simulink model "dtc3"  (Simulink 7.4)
settings: Solver=ode45  StartTime=0.0  StopTime=2  MaxStep=5e-6  RelTol=1e-3
InitFcn:
  | warning off; wmo=0.9 %initial speed
  | fso=1.0 %initial stator flux
undefined symbols (not defined in the file or in its folder): a, wmo

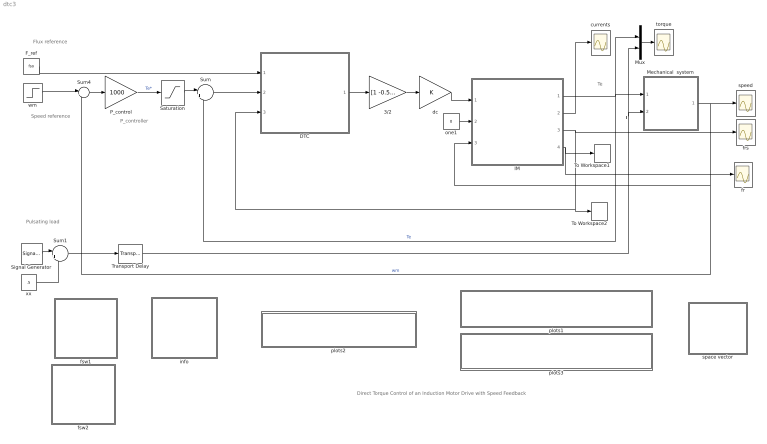
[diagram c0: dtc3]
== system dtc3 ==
  note: Direct Torque Control of an Induction Motor Drive with Speed Feedback
  note: Flux reference
  note: Speed reference
  note: Te
  note: Tl
  note: Pulsating load
  note: P_controller
  3/2 : Gain  Gain=[1 -0.5 -0.5;0 sqrt(3)/2 -sqrt(3)/2]  Multiplication=Matrix(K*u)  ParameterDataType=sfix(16)  ParameterScaling=2^0  OutDataType=sfix(16)  OutScaling=2^0
  DTC : Subsystem
  F_ref : Constant  Value=fso  OutDataType=sfix(16)  OutScaling=2^0
  IM : Subsystem  mask{Rs=0.01, Rr=0.02, Lsl=0.10, Lrl=0.10, Lm=4.5, wo=2*pi*60}
      mask prompts: Rs "Stator resistance [pu]"; Rr "Rotor resistance [pu]"; Lsl "Stator leakage inductance [pu]"; Lrl "Rotor leakage inductance [pu]"; Lm "Magnetizing inductance [pu]"; wo "Base frequency [rad/s]"
  Mechanical  system : Subsystem  mask{H=0.5, Bm=1e-5}
      mask prompts: H "Inertia constant [s]"; Bm "Torque-speed coefficient"
  Mux : Mux  Inputs=2
  P_control : Gain  Gain=1000  ParameterDataType=sfix(16)  ParameterScaling=2^0  OutDataType=sfix(16)  OutScaling=2^0
  Saturation : Saturate  UpperLimit=2  LowerLimit=-2
  Signal Generator : SignalGenerator  WaveForm=square  Amplitude=.5  Frequency=4
  Sum : Sum  Inputs=|+-  OutDataType=sfix(16)  OutScaling=2^0
  Sum1 : Sum  Inputs=|++  OutDataType=sfix(16)  OutScaling=2^0
  Sum4 : Sum  Inputs=|+-  OutDataType=sfix(16)  OutScaling=2^0
  To Workspace1 : ToWorkspace  VariableName=fr  SampleTime=-1  SaveFormat=Array
  To Workspace2 : ToWorkspace  VariableName=fs  SampleTime=-1  SaveFormat=Array
  Transport Delay : TransportDelay  DelayTime=.75
  currents : Scope
  dc : Gain  ParameterDataType=sfix(16)  ParameterScaling=2^0  OutDataType=sfix(16)  OutScaling=2^0
  fr : Scope
  frs : Scope
  fsw1 : Subsystem
  fsw2 : Subsystem
  info : Subsystem
  one1 : Constant  Value=0  OutDataType=sfix(16)  OutScaling=2^0
  plots1 : Subsystem
  plots2 : Subsystem
  plots3 : Subsystem
  space vector : Subsystem
  speed : Scope
  torque : Scope
  wm : Step  Time=.25  Before=wmo  After=.5  SampleTime=0
  xx : Constant  Value=.5  OutDataType=sfix(16)  OutScaling=2^0
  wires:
  DTC/1(s3) -> 3/2/1
  F_ref/1 -> DTC/1(f_ref)
  3/2/1 -> dc/1
  IM/3(fs) -> To Workspace2/1, DTC/3(fs), frs/1
  one1/1 -> IM/2(wk)
  IM/1(Te) -> Mechanical  system/1(Te), Sum/2, Mux/1  "Te"
  Mechanical  system/1(wm) -> speed/1, IM/3(wm), Sum4/2  "wm"
  IM/2(is) -> currents/1
  wm/1 -> Sum4/1
  Sum/1 -> DTC/2(T_er)
  Mux/1 -> torque/1
  Sum4/1 -> P_control/1
  P_control/1 -> Saturation/1  "Te*"
  IM/4(fr) -> To Workspace1/1, fr/1
  dc/1 -> IM/1(vs)
  Signal Generator/1 -> Sum1/1
  xx/1 -> Sum1/2
  Sum1/1 -> Transport Delay/1
  Transport Delay/1 -> Mux/2, Mechanical  system/2(Tl)
  Saturation/1 -> Sum/1

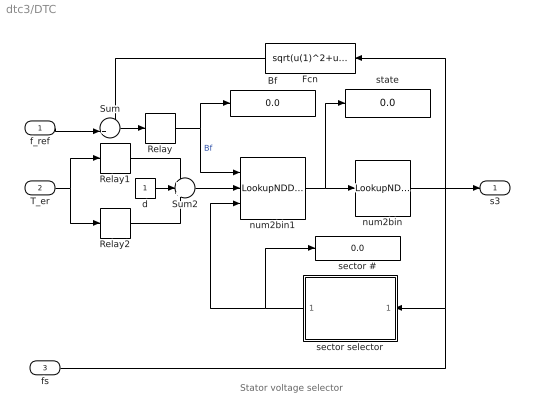
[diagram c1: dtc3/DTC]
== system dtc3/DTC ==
  note: Stator voltage selector
  f_ref : Inport  OutDataType=sfix(16)  OutScaling=2^0
  T_er : Inport  Port=2  OutDataType=sfix(16)  OutScaling=2^0
  fs : Inport  Port=3  OutDataType=sfix(16)  OutScaling=2^0
  Bf : Display
  Fcn : Fcn  Expr=sqrt(u(1)^2+u(2)^2)
  Relay : Relay  OnSwitchValue=.01  OffSwitchValue=-.01  OutDataType=sfix(16)  OutScaling=2^0
  Relay1 : Relay  OnSwitchValue=.02  OffSwitchValue=0  OutDataType=sfix(16)  OutScaling=2^0
  Relay2 : Relay  OnSwitchValue=0  OffSwitchValue=-.02  OnOutputValue=0  OffOutputValue=-1  OutDataType=sfix(16)  OutScaling=2^0
  Sum : Sum  Inputs=-+|  OutDataType=sfix(16)  OutScaling=2^0
  Sum2 : Sum  Inputs=+++  OutDataType=sfix(16)  OutScaling=2^0
  d : Constant  OutDataType=sfix(16)  OutScaling=2^0
  num2bin : LookupNDDirect  InputsSelectThisObjectFromTable=Column  Table=[0 0 0;1 0 0;0 1 0;1 1 0;0 0 1;1 0 1;0 1 1;1 1 1]'  ActionForOutOfRangeInput=Error
  num2bin1 : LookupNDDirect  NumberOfTableDimensions=3  Table=a  ActionForOutOfRangeInput=Error
  sector # : Display
  sector selector : Subsystem
  state : Display
  s3 : Outport
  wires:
  num2bin1/1 -> state/1, num2bin/1
  Sum/1 -> Relay/1
  Relay/1 -> Bf/1, num2bin1/1  "Bf"
  Fcn/1 -> Sum/1
  Sum2/1 -> num2bin1/2
  Relay1/1 -> Sum2/1
  Relay2/1 -> Sum2/3
  d/1 -> Sum2/2
  T_er/1 -> Relay2/1, Relay1/1
  f_ref/1 -> Sum/2
  num2bin/1 -> s3/1
  fs/1 -> Fcn/1, sector selector/1(fs)
  sector selector/1(sector) -> num2bin1/3, sector #/1

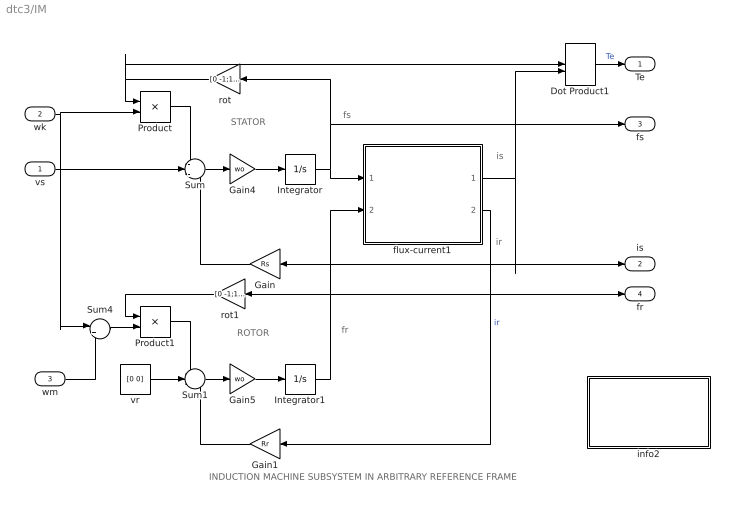
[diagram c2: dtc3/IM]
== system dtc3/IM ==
  note: ROTOR
  note: STATOR
  note: fs
  note: fr
  note: is
  note: INDUCTION MACHINE SUBSYSTEM IN ARBITRARY REFERENCE FRAME
  note: ir
  vs : Inport  OutDataType=sfix(16)  OutScaling=2^0
  wk : Inport  Port=2  OutDataType=sfix(16)  OutScaling=2^0
  wm : Inport  Port=3  OutDataType=sfix(16)  OutScaling=2^0
  Dot Product1 : DotProduct  OutDataType=fixdt(1, 16)  OutScaling=2^-10
  Gain : Gain  Gain=Rs  ParameterDataType=sfix(16)  ParameterScaling=2^0  OutDataType=sfix(16)  OutScaling=2^0
  Gain1 : Gain  Gain=Rr  ParameterDataType=sfix(16)  ParameterScaling=2^0  OutDataType=sfix(16)  OutScaling=2^0
  Gain4 : Gain  Gain=wo  ParameterDataType=sfix(16)  ParameterScaling=2^0  OutDataType=sfix(16)  OutScaling=2^0
  Gain5 : Gain  Gain=wo  ParameterDataType=sfix(16)  ParameterScaling=2^0  OutDataType=sfix(16)  OutScaling=2^0
  Integrator : Integrator  InitialCondition=[fso 0]
  Integrator1 : Integrator  InitialCondition=[1 0]
  Product : Product  OutDataType=sfix(16)  OutScaling=2^0
  Product1 : Product  OutDataType=sfix(16)  OutScaling=2^0
  Sum : Sum  Inputs=-+-  OutDataType=sfix(16)  OutScaling=2^0
  Sum1 : Sum  Inputs=-+-  OutDataType=sfix(16)  OutScaling=2^0
  Sum4 : Sum  Inputs=|+-  OutDataType=sfix(16)  OutScaling=2^0
  flux-current1 : Subsystem
  info2 : Subsystem
  rot : Gain  Gain=[0 -1;1 0]  Multiplication=Matrix(K*u)  ParameterDataType=sfix(16)  ParameterScaling=2^0  OutDataType=sfix(16)  OutScaling=2^0
  rot1 : Gain  Gain=[0 -1;1 0]  Multiplication=Matrix(K*u)  ParameterDataType=sfix(16)  ParameterScaling=2^0  OutDataType=sfix(16)  OutScaling=2^0
  vr : Constant  Value=[0 0]  OutDataType=sfix(16)  OutScaling=2^0
  Te : Outport
  is : Outport  Port=2
  fs : Outport  Port=3
  fr : Outport  Port=4
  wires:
  Gain/1 -> Sum/3
  vr/1 -> Sum1/2
  Gain1/1 -> Sum1/3
  flux-current1/2(ir) -> Gain1/1  "ir"
  Integrator/1 -> flux-current1/1(fs), rot/1, fs/1
  Integrator1/1 -> flux-current1/2(fr), rot1/1, fr/1
  Product1/1 -> Sum1/1
  rot1/1 -> Product1/1
  Product/1 -> Sum/1
  rot/1 -> Product/1, Dot Product1/1
  Sum4/1 -> Product1/2
  Sum/1 -> Gain4/1
  Gain4/1 -> Integrator/1
  Sum1/1 -> Gain5/1
  Gain5/1 -> Integrator1/1
  flux-current1/1(is) -> Gain/1, is/1, Dot Product1/2
  Dot Product1/1 -> Te/1  "Te"
  vs/1 -> Sum/2
  wk/1 -> Product/2, Sum4/1
  wm/1 -> Sum4/2

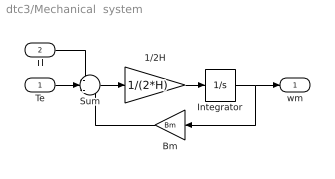
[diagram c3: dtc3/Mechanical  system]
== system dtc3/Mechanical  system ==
  Te : Inport  OutDataType=sfix(16)  OutScaling=2^0
  Tl : Inport  Port=2  OutDataType=sfix(16)  OutScaling=2^0
  1/2H : Gain  Gain=1/(2*H)  ParameterDataType=sfix(16)  ParameterScaling=2^0  OutDataType=sfix(16)  OutScaling=2^0
  Bm : Gain  Gain=Bm  ParameterDataType=sfix(16)  ParameterScaling=2^0  OutDataType=sfix(16)  OutScaling=2^0
  Integrator : Integrator  InitialCondition=wmo
  Sum : Sum  Inputs=-+-  OutDataType=sfix(16)  OutScaling=2^0
  wm : Outport
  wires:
  Tl/1 -> Sum/1
  Te/1 -> Sum/2
  Integrator/1 -> wm/1, Bm/1
  Bm/1 -> Sum/3
  Sum/1 -> 1/2H/1
  1/2H/1 -> Integrator/1

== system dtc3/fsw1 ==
  note: Switching table

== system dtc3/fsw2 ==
  note: Switching table

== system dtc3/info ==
  note: Direct torque control of an induction motordrive
  note: The induction motor operates initially at no load at a speed and a stator flux level specified in a callback of the model properties. The mechanical load torque is initially set at Tl = 0 and the electromagnetic torque Te is set to zero by having stator and rotor space vectors colinear (check the IC's of the flux integrators). Before running, double click the Switching Table block.

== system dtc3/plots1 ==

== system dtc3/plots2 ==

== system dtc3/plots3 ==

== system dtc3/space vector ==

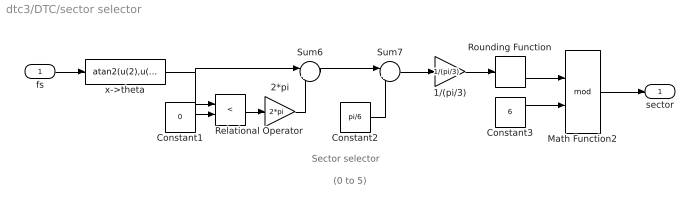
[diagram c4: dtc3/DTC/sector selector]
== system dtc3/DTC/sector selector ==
  note: Sector selector
  note: (0 to 5)
  fs : Inport  OutDataType=sfix(16)  OutScaling=2^0
  1/(pi/3) : Gain  Gain=1/(pi/3)  ParameterDataType=sfix(16)  ParameterScaling=2^0  OutDataType=sfix(16)  OutScaling=2^0
  2*pi : Gain  Gain=2*pi  ParameterDataType=sfix(16)  ParameterScaling=2^0  OutDataType=sfix(16)  OutScaling=2^0
  Constant1 : Constant  Value=0  OutDataType=sfix(16)  OutScaling=2^0
  Constant2 : Constant  Value=pi/6  OutDataType=sfix(16)  OutScaling=2^0
  Constant3 : Constant  Value=6  OutDataType=sfix(16)  OutScaling=2^0
  Math Function2 : Math  Operator=mod
  Relational Operator : RelationalOperator  Operator=<
  Rounding Function : Rounding
  Sum6 : Sum  Inputs=|++  OutDataType=sfix(16)  OutScaling=2^0
  Sum7 : Sum  Inputs=|++  OutDataType=sfix(16)  OutScaling=2^0
  x->theta : Fcn  Expr=atan2(u(2),u(1))
  sector : Outport
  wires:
  Constant1/1 -> Relational Operator/2
  Relational Operator/1 -> 2*pi/1
  2*pi/1 -> Sum6/2
  Sum6/1 -> Sum7/1
  Constant2/1 -> Sum7/2
  Sum7/1 -> 1/(pi/3)/1
  1/(pi/3)/1 -> Rounding Function/1
  Rounding Function/1 -> Math Function2/1
  Constant3/1 -> Math Function2/2
  fs/1 -> x->theta/1
  Math Function2/1 -> sector/1
  x->theta/1 -> Relational Operator/1, Sum6/1

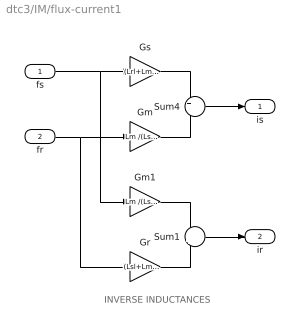
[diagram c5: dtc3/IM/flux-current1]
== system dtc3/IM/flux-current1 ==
  note: INVERSE INDUCTANCES
  fs : Inport  OutDataType=sfix(16)  OutScaling=2^0
  fr : Inport  Port=2  OutDataType=sfix(16)  OutScaling=2^0
  Gm : Gain  Gain=Lm /(Lsl*Lrl+Lsl*Lm+Lrl*Lm)  ParameterDataType=sfix(16)  ParameterScaling=2^0  OutDataType=sfix(16)  OutScaling=2^0
  Gm1 : Gain  Gain=Lm /(Lsl*Lrl+Lsl*Lm+Lrl*Lm)  ParameterDataType=sfix(16)  ParameterScaling=2^0  OutDataType=sfix(16)  OutScaling=2^0
  Gr : Gain  Gain=(Lsl+Lm )/(Lsl*Lrl+Lsl*Lm+Lrl*Lm)  ParameterDataType=sfix(16)  ParameterScaling=2^0  OutDataType=sfix(16)  OutScaling=2^0
  Gs : Gain  Gain=(Lrl+Lm) /(Lsl*Lrl+Lsl*Lm+Lrl*Lm)  ParameterDataType=sfix(16)  ParameterScaling=2^0  OutDataType=sfix(16)  OutScaling=2^0
  Sum1 : Sum  Inputs=-+  OutDataType=sfix(16)  OutScaling=2^0
  Sum4 : Sum  Inputs=+-  OutDataType=sfix(16)  OutScaling=2^0
  is : Outport
  ir : Outport  Port=2
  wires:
  fs/1 -> Gs/1, Gm1/1
  Gs/1 -> Sum4/1
  fr/1 -> Gm/1, Gr/1
  Gm/1 -> Sum4/2
  Sum4/1 -> is/1
  Gm1/1 -> Sum1/1
  Gr/1 -> Sum1/2
  Sum1/1 -> ir/1

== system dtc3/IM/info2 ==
  note: Synchronous machine transients under shortcircuit
  note: This demonstration illustrates the dynamics of a synchronous generator, initially at no load, following a three-phase short circuit at the terminals.
